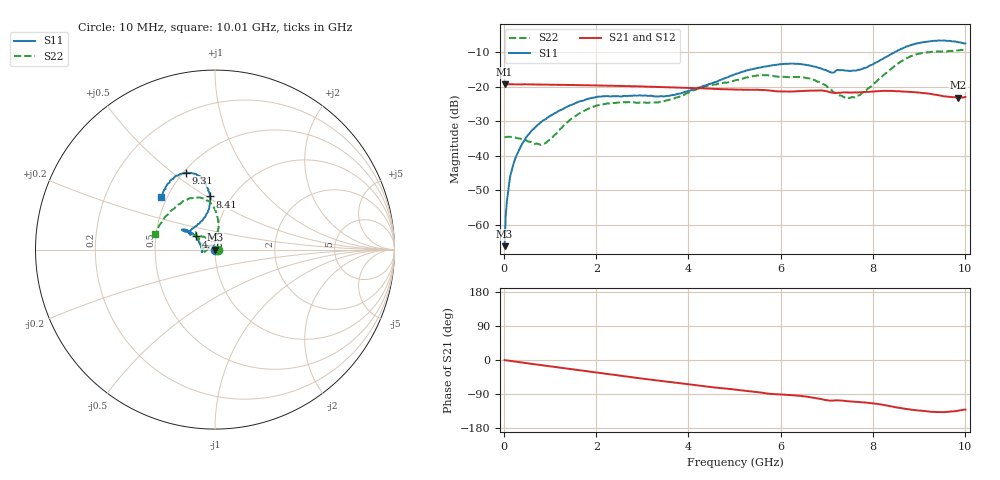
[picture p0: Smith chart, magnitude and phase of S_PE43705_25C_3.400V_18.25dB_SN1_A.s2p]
! Device ID: PE43705
! Serial: 1
! Insertion: A
! Impedance: 50 ohm
! Temp: 25C
! VDD: 3.400V
! Attenuation Step: 18.25dB
#  Hz  S  RI  R  50
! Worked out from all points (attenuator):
!   401 points, 10 MHz to 10.01 GHz, reference 50 ohm
!   highest |S21| = -19.30 dB at 10 MHz (marker M1); lowest = -23.2 dB at 9.86 GHz (marker M2)
!   lowest |S11| = -66.2 dB at 10 MHz (marker M3), VSWR 1.00, Z = 50 + j0.0439 ohm
!   |S11| at or under -10 dB: start of sweep to 8.48 GHz
!   |S22| runs from -36.9 to -9.3 dB; largest |S21 - S12| = 0.0012
!   S11 on the Smith chart (normalised r, x): 10 MHz: 1.00, +0.00; 4.76 GHz: 0.80, +0.12; 8.41 GHz: 0.79, +0.52; 9.31 GHz: 0.51, +0.56; 10.01 GHz: 0.46, +0.33
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1e7  -0.000216 0.000439  0.1083 -0.00046  0.1084 -0.00038  0.0184 0.000241
8.5e7  -1.11e-05 0.00298  0.1079 -0.00293  0.108 -0.0029  0.0187 0.00199
1.6e8  -0.000476 0.00595  0.1079 -0.00539  0.1079 -0.00532  0.0181 0.00423
2.6e8  -0.00177 0.00965  0.1074 -0.00858  0.1073 -0.00851  0.0167 0.00695
4.35e8  -0.00551 0.0155  0.1069 -0.0142  0.1066 -0.0139  0.0131 0.011
8.85e8  -0.0247 0.0223  0.103 -0.0278  0.1031 -0.0276  -0.00533 0.014
1.685e9  -0.0613 0.00927  0.0923 -0.0493  0.0923 -0.0493  -0.043 0.000413
2.26e9  -0.072 -0.00853  0.0817 -0.0625  0.0818 -0.0625  -0.0558 -0.0117
3.36e9  -0.0717 -0.00487  0.0569 -0.0805  0.057 -0.0803  -0.0592 0.00274
4.76e9  -0.1067 0.073  0.024 -0.0883  0.0241 -0.0883  -0.0924 0.0656
5.01e9  -0.1223 0.0881  0.0187 -0.0886  0.0188 -0.0886  -0.0985 0.0739
5.985e9  -0.1778 0.113  -0.00128 -0.0849  -0.000942 -0.085  -0.1055 0.0896
6.685e9  -0.1697 0.101  -0.0137 -0.0863  -0.0137 -0.0862  -0.0991 0.0782
7.11e9  -0.1344 0.0868  -0.0242 -0.0782  -0.024 -0.0782  -0.0559 0.0682
7.535e9  -0.0991 0.1362  -0.0275 -0.0771  -0.027 -0.0772  -0.0118 0.069
7.785e9  -0.0657 0.1697  -0.0306 -0.077  -0.0303 -0.0772  0.00503 0.0821
8.36e9  -0.0261 0.2849  -0.0451 -0.0741  -0.0449 -0.074  0.016 0.172
8.41e9  -0.0292 0.2964  -0.0464 -0.0727  -0.0463 -0.0729  0.013 0.1818
8.86e9  -0.0776 0.3973  -0.055 -0.0624  -0.0542 -0.063  -0.0473 0.275
9.31e9  -0.163 0.428  -0.0561 -0.0525  -0.0563 -0.0528  -0.1499 0.2819
9.86e9  -0.2756 0.3385  -0.0477 -0.0498  -0.0478 -0.0495  -0.2968 0.152
1.001e10  -0.2991 0.2938  -0.046 -0.0534  -0.0466 -0.0532  -0.3327 0.0882
